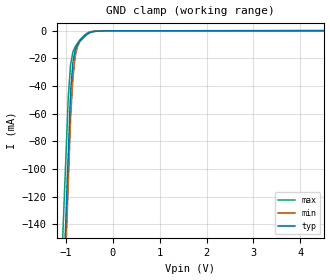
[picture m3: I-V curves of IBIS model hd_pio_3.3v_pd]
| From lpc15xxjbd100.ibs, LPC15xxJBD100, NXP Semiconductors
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[Model] hd_pio_3.3v_pd
Model_type Input
Vinl = 990.000mV
Vinh = 2.31000V
C_comp 1.52000pF 1.52000pF 1.52000pF
| variable typ   min   max
[Voltage Range] 3.30000V 3.00000V 3.60000V
[POWER Clamp Reference] 3.30000V 3.00000V 3.60000V
[GND Clamp Reference] 0.00000V 0.00000V 0.00000V
[Temperature Range]   25   85   -40
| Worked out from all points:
|   GND clamp passes 1 mA (typ) near -0.46 V on its own axis
[GND Clamp]
-3.3V     -2.224A    -2.356A    -2.062A
-950mV    -89.59mA   -111.1mA   -48.37mA
-900mV    -44.18mA   -63.3mA    -24.43mA
-850mV    -22.8mA    -33.98mA   -15.23mA
-800mV    -13.64mA   -18.15mA   -11.36mA
-750mV    -9.681mA   -11.04mA   -8.929mA
-700mV    -7.2mA     -7.752mA   -6.494mA
-600mV    -3.968mA   -4.033mA   -3.033mA
-500mV    -1.419mA   -1.54mA    -916.2uA
-350mV    -377.9uA   -249.4uA   -196.4uA
50mV      -30.72uA   2.936uA    -7.58uA
6.6V      152.4uA    134.8uA    141.8uA
[POWER Clamp]
-3.3V     0A         0A         0A
6.6V      0A         0A         0A
